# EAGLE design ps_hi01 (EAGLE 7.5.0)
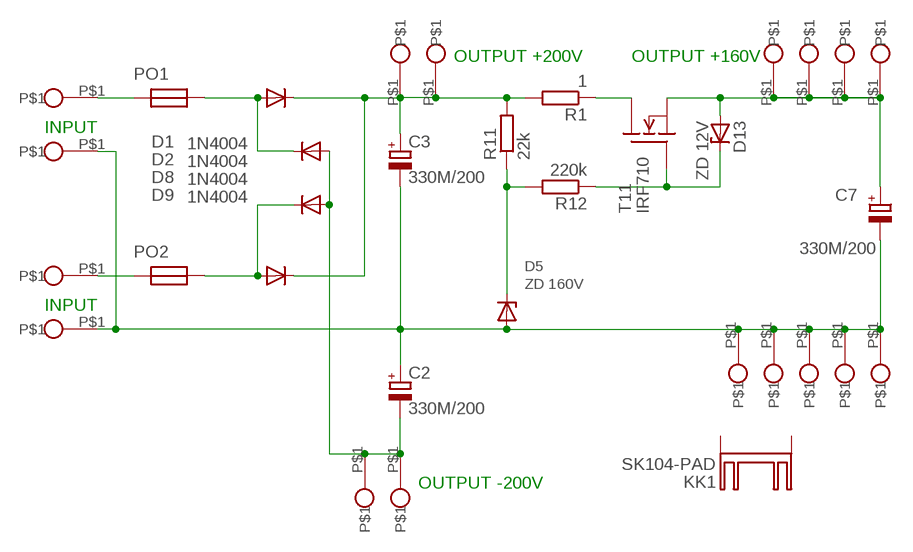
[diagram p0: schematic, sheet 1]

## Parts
C2  330M/200  CPOL-EUE10-22.5  [EB22,5D]
C3  330M/200  CPOL-EUE10-22.5  [EB22,5D]
C7  330M/200  CPOL-EUE10-22.5  [EB22,5D]
D1  1N4004  [DO41-10]
D2  1N4004  [DO41-10]
D5  ZD 160V  BZW03XX  [SOD64Z12]
D8  1N4004  [DO41-10]
D9  1N4004  [DO41-10]
D13  ZD 12V  BZW03XX  [SOD64Z12]
KK1  SK104-PAD  [SK104-PAD]
PO1  POJ520  [POJ_SHH1]
PO2  POJ520  [POJ_SHH1]
R1  1  R-EU_0207/10  [0207/10]
R11  22k  R-EU_0207/10  [0207/10]
R12  220k  R-EU_0207/10  [0207/10]
T11  IRF710  IRF840V  [TO220V]
U$1  PIN  [PIN]
U$2  PIN  [PIN]
U$3  PIN  [PIN]
U$4  PIN  [PIN]
U$5  PIN  [PIN]
U$6  PIN  [PIN]
U$7  PIN  [PIN]
U$8  PIN  [PIN]
U$9  PIN  [PIN]
U$10  PIN  [PIN]
U$11  PIN  [PIN]
U$12  PIN  [PIN]
U$13  PIN  [PIN]
U$14  PIN  [PIN]
U$15  PIN  [PIN]
U$19  PIN  [PIN]
U$20  PIN  [PIN]

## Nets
GND: C2.+ C3.- C7.- D5.A U$1.P$1 U$7.P$1 U$8.P$1 U$9.P$1 U$11.P$1 U$12.P$1 U$13.P$1
N$1: C7.+ D13.A T11.3(S) U$4.P$1 U$5.P$1 U$6.P$1 U$20.P$1
N$2: C2.- D8.A D9.A U$3.P$1 U$14.P$1
N$3: PO2.P$2 U$19.P$1
N$4: PO1.P$2 U$10.P$1
N$5: D2.A D9.C PO2.P$4
N$6: C3.+ D1.C D2.C R1.2 R11.2 U$2.P$1 U$15.P$1
N$7: D5.C R11.1 R12.2
N$8: R1.1 T11.2(D)
N$19: D1.A D8.C PO1.P$4
N$35: D13.C R12.1 T11.1(G)
Unconnected: KK1.K1(K) KK1.K2(K)

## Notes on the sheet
- OUTPUT +200V | OUTPUT +160V
- INPUT
- INPUT
- OUTPUT -200V

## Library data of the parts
C2 C3 C7 = rcl:CPOL-EU: POLARIZED CAPACITOR, European symbol
D1 D2 D8 D9 = diode:1N4004: DIODE
D5 D13 = diode:BZW03XX: Z DIODE
KK1 = heatsink:SK104-PAD: HEATSINK
PO1 PO2 = lampy04:POJ5*20
R1 R11 R12 = rcl:R-EU_: RESISTOR, European symbol
T11 = transistor-fet:IRF840: N-Channel Enhancement MOSFET (HEXFET); 500V; 8A; 0,85Ohm
U$1-U$15 U$19 U$20 = LAMPY02:PIN

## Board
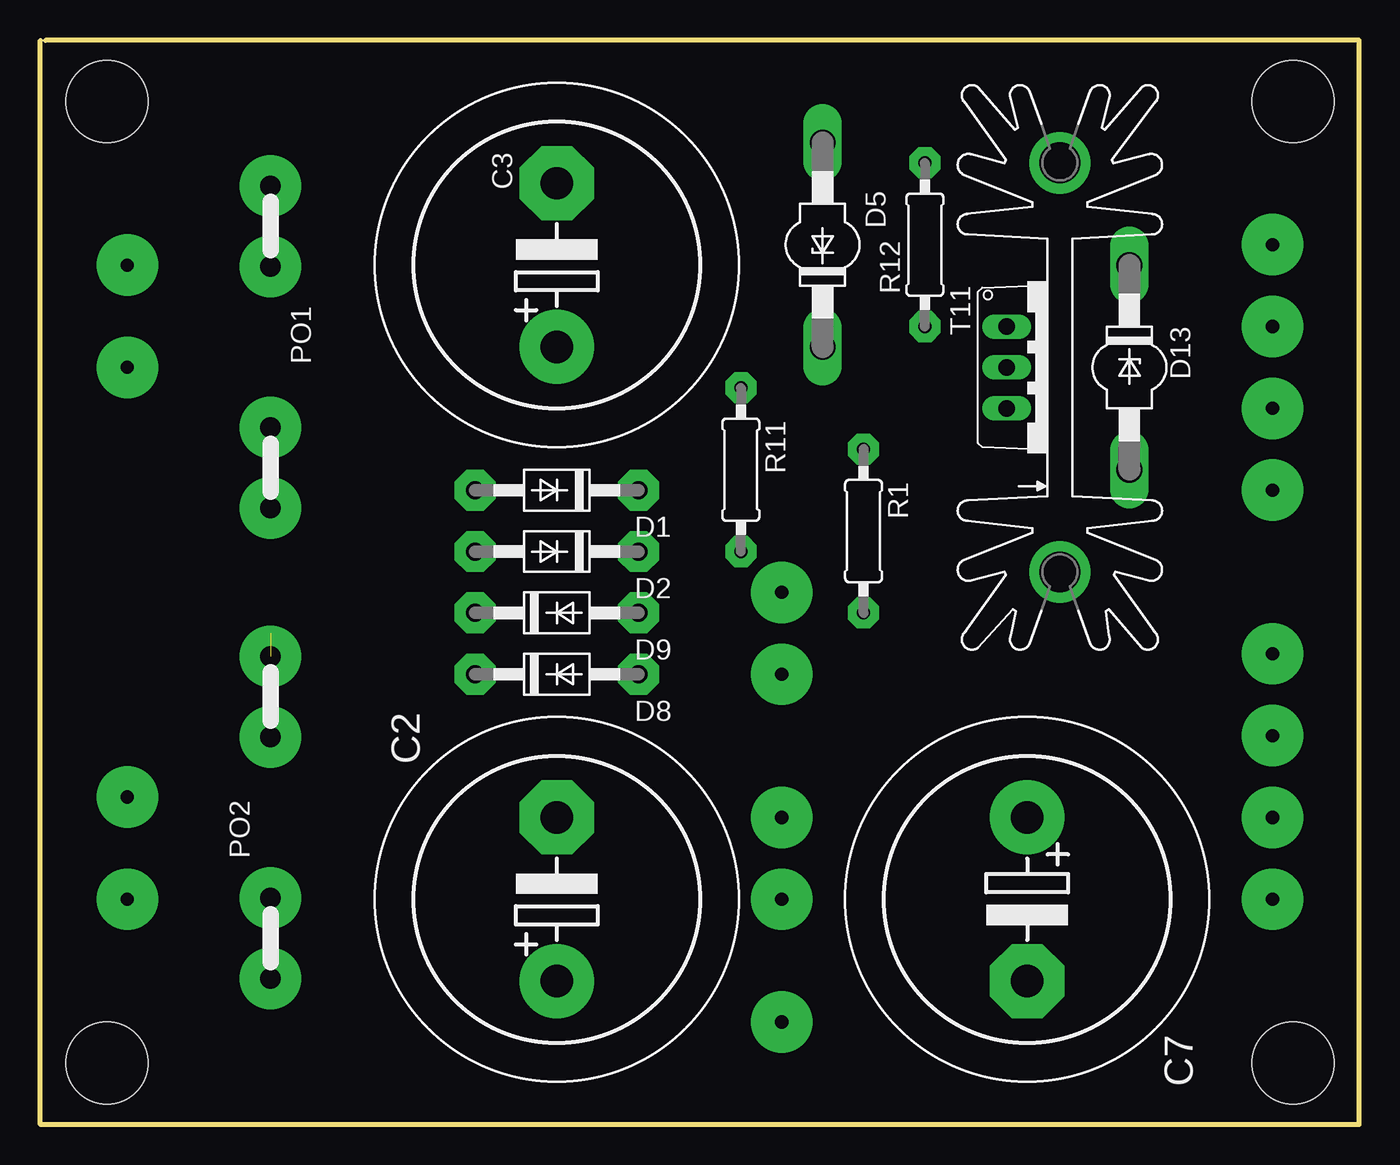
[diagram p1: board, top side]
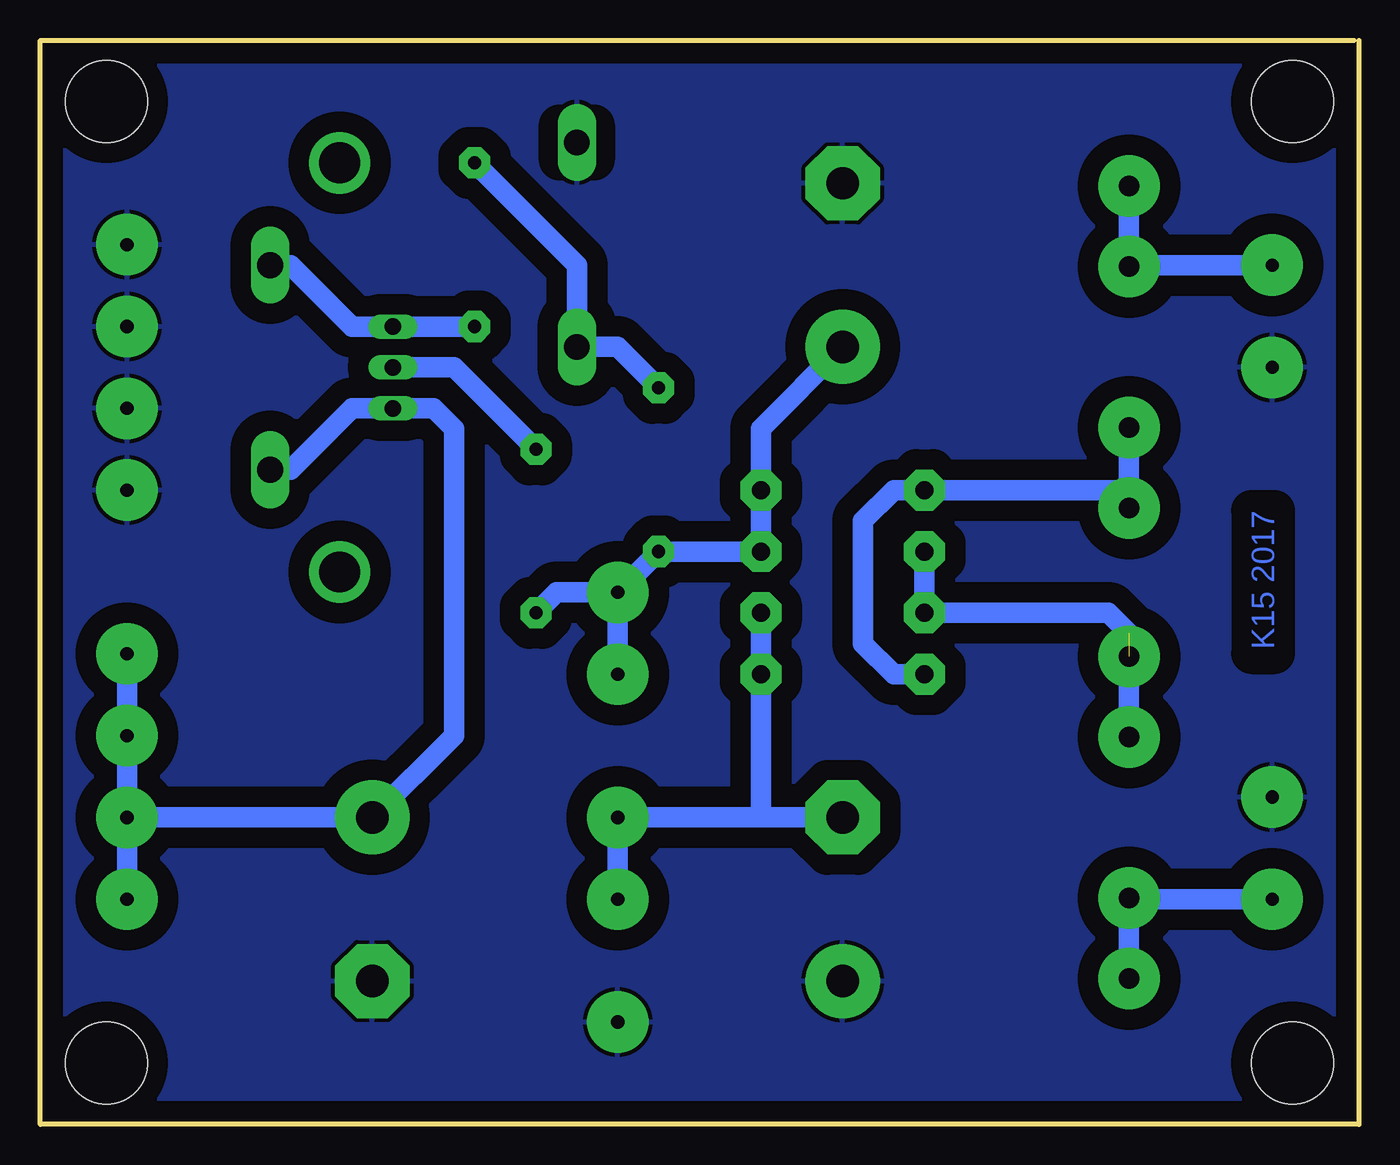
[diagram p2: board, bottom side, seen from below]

Size 81.92 x 67.3 mm. Coordinates in mm from the lower left corner, seen from the top.
Outline: 0.33,67.3 81.92,67.3 81.92,0 0,0 0,67.3
Copper layers (1*16): Top 0.035mm / dielectric 1.5mm / Bottom 0.035mm
Design rules "default": minimum track width 10mil, minimum drill 24mil, track to track 8mil, track to pad 8mil, pad to pad 8mil, via to via 8mil, smd to smd 8mil, copper to edge 40mil, drill to drill 8mil, minimum pad ring 10mil, minimum via ring 8mil, stop-mask expansion 4mil, vias tented up to drill 0mil, thermal gap 10mil
Holes 5.08 mm at 4.14,3.81 77.8,3.81 4.14,63.5 77.8,63.5

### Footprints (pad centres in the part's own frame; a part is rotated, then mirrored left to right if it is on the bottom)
EB22,5D = drill 2.007 pad 4.597: + -5.08,0 | drill 2.007 pad 4.597 octagon: - 5.08,0
DO41-10 = drill 1.118 pad 2.54 octagon: A 5.08,0; C -5.08,0
SOD64Z12 = drill 1.6 long: A 6.35,0; C -6.35,0
SK104-PAD = drill 2.54 pad 3.81: K1 -12.7,-0.762; K2 12.7,-0.762
POJ_SHH1 = drill 1.27 pad 3.81: P$1 -5,0; P$2 -10,0; P$3 5,0; P$4 10,0
0207/10 = drill 0.813 pad 1.93 octagon: 1 -5.08,0; 2 5.08,0
TO220V = drill 1.016 long: 1 -2.54,-2.54; 2 0,-2.54; 3 2.54,-2.54
PIN = drill 0.813 pad 3.81: P$1 0,0

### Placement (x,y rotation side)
C2  32.08,13.97 90 top
C3  32.08,53.34 90 top
C7  61.29,13.97 270 top
D1  32.08,39.37 180 top
D2  32.08,35.56 180 top
D5  48.59,54.61 90 top
D8  32.08,27.94 0 top
D9  32.08,31.75 0 top
D13  67.64,46.99 270 top
KK1  62.56,46.99 90 top
PO1  14.3,48.26 270 top
PO2  14.3,19.05 90 top
R1  51.13,36.83 270 top
R11  43.51,40.64 270 top
R12  54.94,54.61 90 top
T11  62.56,46.99 270 top
U$1  5.41,46.99 0 top
U$2  46.05,33.02 0 top
U$3  46.05,13.97 0 top
U$4  76.53,19.05 0 top
U$5  76.53,24.13 0 top
U$6  76.53,29.21 0 top
U$7  46.05,6.35 0 top
U$8  76.53,44.45 0 top
U$9  5.41,20.32 0 top
U$10  5.41,53.34 90 top
U$11  76.53,39.37 0 top
U$12  76.53,54.61 0 top
U$13  76.53,49.53 0 top
U$14  46.05,19.05 0 top
U$15  46.05,27.94 0 top
U$19  5.41,13.97 90 top
U$20  76.53,13.97 0 top

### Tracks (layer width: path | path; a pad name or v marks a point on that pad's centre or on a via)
GND
  pour Bottom (isolate 1.27): 0.33,67.31 81.61,67.31 81.61,0 0.33,0
N$1
  Bottom 1.27: U$4.P$1 C7.+ 56.21,24.13 56.21,43.18 57.48,44.45 T11.3 62.56,44.45 66.37,40.64 D13.A | U$4.P$1 U$5.P$1 U$6.P$1 | U$20.P$1 U$4.P$1
N$2
  Bottom 1.27: D9.A D8.A 37.16,19.05 | C2.- 37.16,19.05 | 37.16,19.05 U$14.P$1 U$3.P$1
N$3
  Bottom 1.27: PO2.P$2 14.3,13.97 U$19.P$1
N$4
  Bottom 1.27: PO1.P$2 14.3,53.34 U$10.P$1
N$5  (1 unrouted)
  Bottom 1.27: 14.3,24.13 14.3,30.48 15.57,31.75 D9.C D2.A
N$6
  Bottom 1.27: C3.+ 37.16,43.18 D1.C D2.C R11.2 U$2.P$1 | U$2.P$1 U$15.P$1 | R1.2 49.86,33.02 U$2.P$1
N$7
  Bottom 1.27: R11.1 46.05,48.26 D5.C 48.59,53.34 R12.2
N$8
  Bottom 1.27: T11.2 56.21,46.99 R1.1
N$9  (via drill 0.6 pad 2.18)
  other vias: 48.59,48.26
N$10  (via drill 0.6 pad 2.18)
  other vias: 48.59,60.96
N$11  (via drill 0.6 pad 2.18)
  other vias: 67.64,53.34
N$12  (via drill 0.6 pad 2.18)
  other vias: 67.64,40.64
N$19
  Bottom 1.27: D8.C 28.91,27.94 30.81,29.84 30.81,37.47 28.91,39.37 D1.A 14.3,39.37 | 14.3,39.37 PO1.P$4 | 14.3,43.18 14.3,39.37
N$35
  Bottom 1.27: R12.1 T11.1 62.56,49.53 66.37,53.34 D13.C

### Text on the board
Bottom: K15 2017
